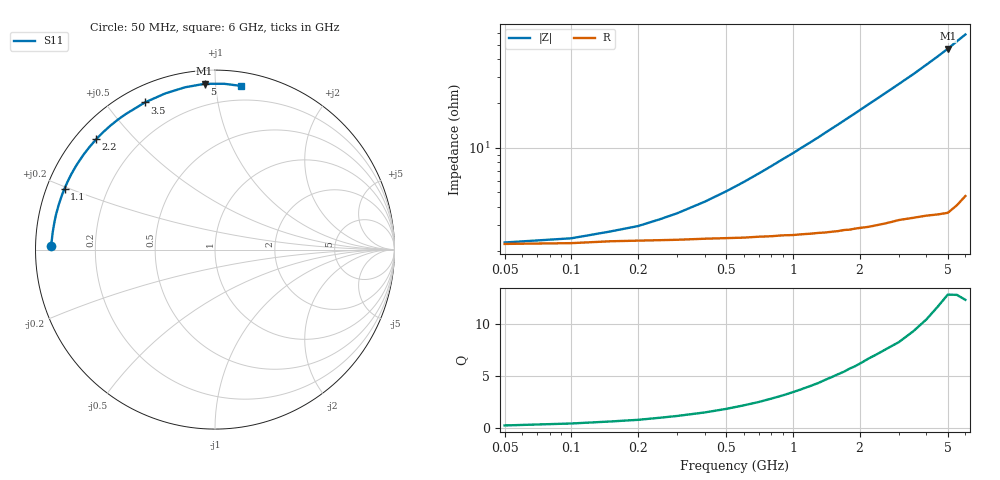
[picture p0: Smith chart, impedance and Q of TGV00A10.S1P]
! SIEMENS Discrete & RF Semiconductors
! BAT64
! Si Schottky Diode in SOT23
! IF = 100 mA
! S-Parameters:  February  1997
# GHz  S  MA  R  50
!  f  S11
! GHz  MAG  ANG
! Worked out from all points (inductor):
!   34 points, 50 MHz to 6 GHz, reference 50 ohm
!   read as one part to ground: L = 1.41 nH near 900 MHz
!   highest Q = 12.9 at 5 GHz (marker M1), where L = 1.49 nH
!   S11 on the Smith chart (normalised r, x): 50 MHz: 0.04, +0.01; 1.1 GHz: 0.05, +0.19; 2.2 GHz: 0.06, +0.39; 3.5 GHz: 0.07, +0.63; 5 GHz: 0.07, +0.94; 6 GHz: 0.09, +1.17
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0.05  0.9144 178.9
0.1  0.9134 177.9
0.15  0.911 176.8
0.2  0.9102 175.9
0.25  0.9097 174.8
0.5  0.9074 169.8
0.6  0.907 167.8
0.8  0.9058 163.8
0.9  0.9051 161.8
1  0.9051 159.9
1.1  0.9046 157.9
1.3  0.904 154.1
1.4  0.9041 152.1
1.6  0.9038 148.3
1.8  0.9035 144.5
1.9  0.9031 142.7
2  0.9031 140.8
2.2  0.9036 137.1
2.4  0.9035 133.6
2.6  0.9037 130.1
2.8  0.904 126.7
3  0.9042 123.4
3.5  0.9082 115.5
4  0.9132 107.7
4.5  0.9196 100.5
5  0.9256 93.6
5.5  0.9253 86.9
6  0.9234 80.9
